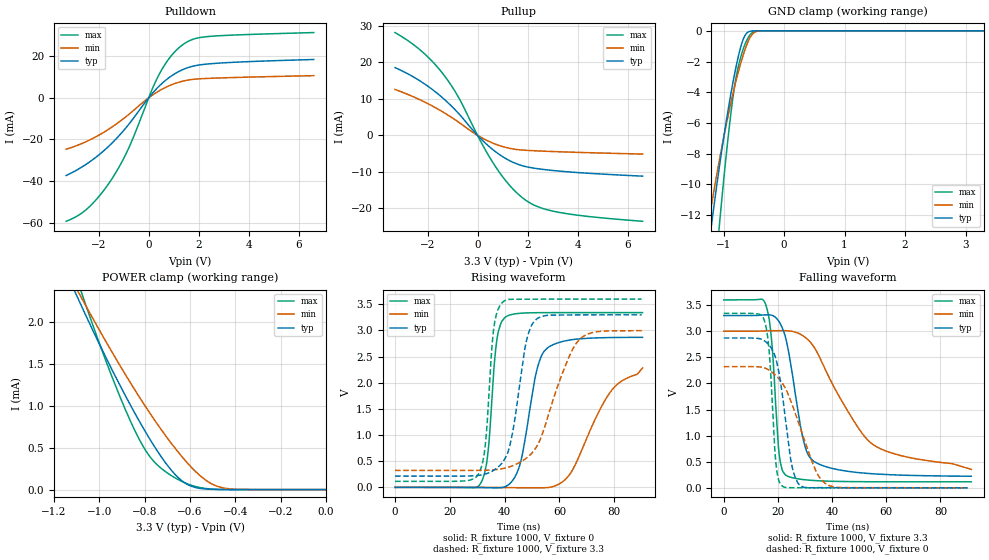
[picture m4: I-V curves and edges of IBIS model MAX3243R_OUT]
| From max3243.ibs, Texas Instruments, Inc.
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[Model]   MAX3243R_OUT
Model_type  3-state
Enable   Active-High
Vref =   0.0
Rref =   3000
Cref =   150p
Vmeas =   1.5
| variable   typ   min   max
C_comp   2.23pF   1.86pF   2.43pF
| C_pullup   2.87pF   2.10pF   4.07pF
| C_pulldown   3.15pF   2.18pF   4.52pF
| C_tri-state   2.23pF   1.86pF   2.43pF
[Temperature Range]   40   100   -40
| Ambient temperature   25   85   -40
[Voltage range]   3.3   3   3.6
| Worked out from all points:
|   slope of the pulldown table from 0 to 0.495 V, typ, clamps not added: 75.9 ohm
|   slope of the pullup table from 0 to 0.495 V, typ, clamps not added: 152 ohm
|   GND clamp passes 1 mA (typ) near -0.71 V on its own axis
|   POWER clamp passes 1 mA (typ) near -0.86 V on its own axis
|   rising waveform, R_fixture 1000, V_fixture 0: 20-80 % time 5.78ns typ, 12.6ns min, 2.89ns max; typ from 0 V to 2.87 V
|   falling waveform, R_fixture 1000, V_fixture 3.3: 20-80 % time 6.14ns typ, 18.2ns min, 2.63ns max; typ from 3.3 V to 0.222 V
|   rising waveform, R_fixture 1000, V_fixture 3.3: 20-80 % time 5.47ns typ, 10.7ns min, 2.8ns max; typ from 0.215 V to 3.3 V
|   falling waveform, R_fixture 1000, V_fixture 0: 20-80 % time 4.6ns typ, 9.67ns min, 2.28ns max; typ from 2.87 V to 0 V
[GND Clamp]
| MAX3243R_OUT_33
|   Voltage   I(typ)   I(min)   I(max)
-3.3V     -112.7mA   -87.54mA   -165.5mA
-1.28V    -15.19mA   -13.29mA   -22.6mA
-1.245V   -14.07mA   -12.44mA   -20.85mA
-1.195V   -12.52mA   -11.25mA   -18.42mA
-1.085V   -9.312mA   -8.783mA   -13.38mA
-1.055V   -8.486mA   -8.141mA   -12.09mA
-910mV    -4.823mA   -5.262mA   -6.45mA
-815mV    -2.767mA   -3.604mA   -3.55mA
-695mV    -781.3uA   -1.837mA   -1.438mA
-590mV    -70.41uA   -662uA     -427.4uA
-395mV    -103.5nA   -6.484uA   -967.5nA
3.3V      6.8pA      195.1nA    6.312pA
[POWER Clamp]
| MAX3243R_OUT_33
|   Voltage   I(typ)   I(min)   I(max)
-3.3V     21.3mA     17.42mA    29.07mA
-1.11V    2.383mA    2.45mA     2.613mA
-1.075V   2.175mA    2.275mA    2.33mA
-940mV    1.413mA    1.627mA    1.322mA
-860mV    997.5uA    1.265mA    804uA
-795mV    685.2uA    988.4uA    466.1uA
-725mV    385.5uA    710.4uA    249.9uA
-670mV    193.6uA    509.9uA    147uA
-615mV    67.26uA    329.2uA    72.73uA
-490mV    2.211uA    49.99uA    4.226uA
-390mV    113.1nA    3.133uA    131.3nA
-48.03fV  6.8pA      37.29pA    7.219pA
[Pulldown]
| MAX3243R_OUT_33
|   Voltage   I(typ)   I(min)   I(max)
-3.3V     -37.35mA   -24.71mA   -59.38mA
-2.41V    -31.22mA   -20.55mA   -52.79mA
-1.945V   -26.98mA   -17.62mA   -46.77mA
-1.49V    -22.02mA   -14.21mA   -39.29mA
-790mV    -12.63mA   -7.934mA   -23.9mA
105mV     1.553mA    924uA      3.189mA
405mV     5.483mA    3.267mA    10.97mA
845mV     9.985mA    5.942mA    19.36mA
1.325V    13.36mA    7.893mA    25.21mA
1.77V     15.21mA    8.872mA    28.15mA
2.345V    16.25mA    9.321mA    29.43mA
6.6V      18.42mA    10.64mA    31.37mA
[Pullup]
| MAX3243R_OUT_33
|   Voltage   I(typ)   I(min)   I(max)
-3.3V     18.59mA    12.58mA    28.2mA
-2.245V   14.69mA    9.568mA    23.13mA
-1.79V    12.49mA    7.978mA    20.15mA
-1.375V   10.15mA    6.357mA    16.82mA
-760mV    6.019mA    3.628mA    10.43mA
130mV     -924.9uA   -518.6uA   -1.72mA
660mV     -4.185mA   -2.269mA   -7.977mA
1.255V    -6.853mA   -3.532mA   -13.52mA
1.84V     -8.438mA   -4.072mA   -17.38mA
2.415V    -9.176mA   -4.283mA   -19.61mA
3.215V    -9.787mA   -4.504mA   -21.09mA
6.6V      -11.21mA   -5.144mA   -23.6mA
[Ramp]
| MAX3243R_OUT_33
| variable   typ   min   max
dV/dt_r   1.73/6.06E-09   1.32/1.19E-08   2.01/2.99E-09
dV/dt_f   1.85/6.38E-09   1.54/1.72E-08   2.10/2.70E-09
R_load = 1000
[Rising Waveform]
| MAX3243R_OUT_33
R_fixture =   1000
C_fixture =   0
L_fixture =   0
V_fixture =   0
V_fixture_min = 0
V_fixture_max = 0
|   Time   V(typ)   V(min)   V(max)
0s        -701.7nV   -1.386uV   -227.6nV
31.14ns   -3.563mV   -361.1uV   69.01mV
33.82ns   -6.895mV   -986.9uV   621.4mV
37.23ns   -9.116mV   -2.406mV   2.843V
40.32ns   17.08mV    -4.651mV   3.259V
45.51ns   419.9mV    -7.296mV   3.329V
54.5ns    2.607V     -8.048mV   3.341V
62.93ns   2.81V      194.7mV    3.342V
78.3ns    2.865V     1.805V     3.342V
90.32ns   2.869V     2.285V     3.342V
[Falling Waveform]
| MAX3243R_OUT_33
R_fixture =   1000
C_fixture =   0
L_fixture =   0
V_fixture =   3.3
V_fixture_min = 3
V_fixture_max = 3.6
|   Time   V(typ)   V(min)   V(max)
0s        3.3V       3V         3.6V
15.51ns   3.313V     3.006V     3.506V
17.75ns   3.305V     3.009V     2.77V
20.47ns   3.179V     3.01V      638mV
22.83ns   2.874V     3.01V      244.1mV
29.17ns   966.5mV    2.915V     159.7mV
33.27ns   506.9mV    2.7V       140.7mV
45.45ns   319.4mV    1.498V     120.9mV
54.67ns   270.9mV    847.2mV    117.2mV
91.43ns   222.5mV    353.1mV    115.3mV
[Rising Waveform]
| MAX3243R_OUT_33
R_fixture =   1000
C_fixture =   0
L_fixture =   0
V_fixture =   3.3
V_fixture_min = 3
V_fixture_max = 3.6
|   Time   V(typ)   V(min)   V(max)
0s        215.4mV    323.9mV    115.2mV
30.33ns   228.5mV    324.3mV    242.4mV
32.88ns   253.9mV    327.1mV    783.3mV
36.2ns    333.1mV    336.9mV    3.101V
39.69ns   512.9mV    363.1mV    3.56V
42.88ns   1.044V     412.9mV    3.597V
47.94ns   2.797V     560.3mV    3.599V
51.31ns   3.201V     749.5mV    3.599V
66.84ns   3.298V     2.801V     3.6V
90ns      3.3V       2.997V     3.6V
[Falling Waveform]
| MAX3243R_OUT_33
R_fixture =   1000
C_fixture =   0
L_fixture =   0
V_fixture =   0
V_fixture_min = 0
V_fixture_max = 0
|   Time   V(typ)   V(min)   V(max)
0s        2.87V      2.321V     3.342V
14.96ns   2.818V     2.298V     3.207V
16.77ns   2.733V     2.253V     2.611V
19.36ns   2.447V     2.146V     420mV
21.83ns   1.707V     1.988V     24.81mV
25.31ns   390.5mV    1.585V     2.975mV
29.2ns    18.41mV    1.005V     1.906mV
34.52ns   3.755mV    271.2mV    1.04mV
39.45ns   2.762mV    33.94mV    593.4uV
90ns      148.3uV    927.8uV    3.623uV
